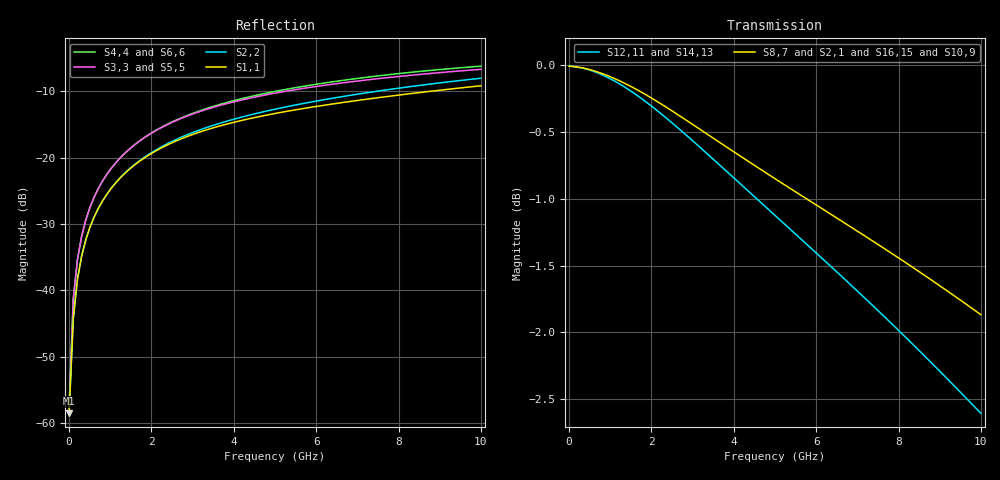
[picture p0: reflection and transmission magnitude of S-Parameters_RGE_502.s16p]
! Touchstone file written by nWave 4.6.3
! Mon Mar 11 11:23:30 2013
! Nimbic
! Project: arc_modified
! Simulation: WAVE1
! User: a0220810
! Computer: dflcmp3924.dal.design.ti.com
! Single-ended  S-parameters
!NUMBER OF PORTS = 16
!  PORT#  PORT_NAME  NET_NAME
! PORT1:  11_BONDWIRE0.PIN020_GND 11
! PORT2:  11_Bot.PIN029_GND 11
! PORT3:  12_BONDWIRE0.PIN021_GND 12
! PORT4:  12_Bot.PIN028_GND 12
! PORT5:  19_BONDWIRE0.PIN012_GND 19
! PORT6:  19_Bot.PIN023_GND 19
! PORT7:  20_BONDWIRE0.PIN007_GND 20
! PORT8:  20_Bot.PIN024_GND 20
! PORT9:  22_BONDWIRE0.PIN009_GND 22
! PORT10:  22_Bot.PIN026_GND 22
! PORT11:  23_BONDWIRE0.PIN010_GND 23
! PORT12:  23_Bot.PIN027_GND 23
! PORT13:  8_BONDWIRE0.PIN018_GND 8
! PORT14:  8_Bot.PIN032_GND 8
! PORT15:  9_BONDWIRE0.PIN022_GND 9
! PORT16:  9_Bot.PIN031_GND 9
# HZ S RI R 50
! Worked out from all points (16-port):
!   100 points, 100 Hz to 10 GHz, reference 50 ohm
!   strongest paths, dB at 100 Hz, 2.525 GHz, 5.051 GHz, 7.576 GHz, 10 GHz:
!     S8,7: 0.0, -0.3, -0.9, -1.4, -1.9
!     S2,1: 0.0, -0.4, -0.9, -1.4, -1.9
!     S16,15: 0.0, -0.4, -0.9, -1.4, -2.0
!     S10,9: 0.0, -0.4, -0.9, -1.5, -2.0
!     S12,11: 0.0, -0.4, -1.1, -1.9, -2.6
!     S14,13: 0.0, -0.4, -1.2, -1.9, -2.7
!   lowest |S11| = -58.6 dB at 100 Hz (marker M1), VSWR 1.00, Z = 50.1 + j6.45e-07 ohm
!   |S11| at or under -10 dB: start of sweep to 8.796 GHz
